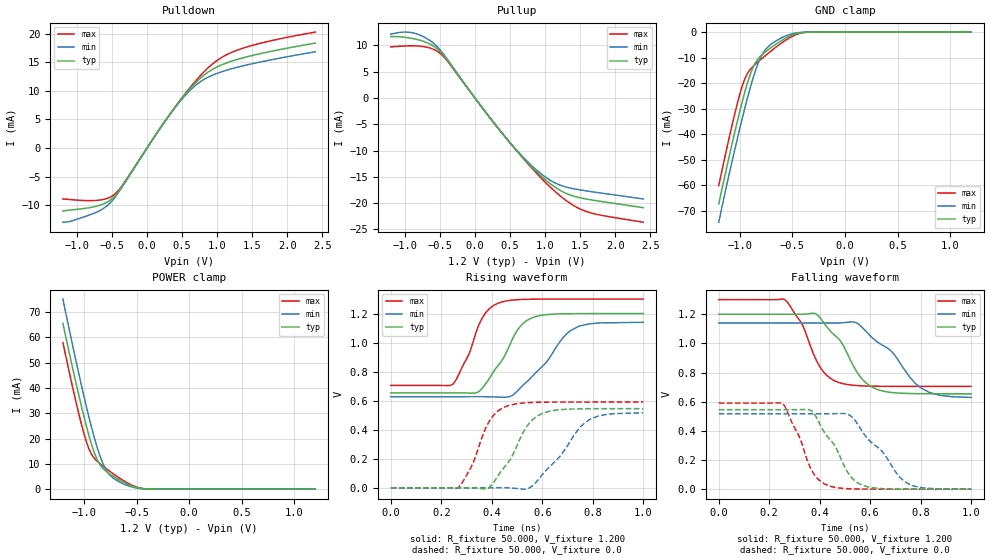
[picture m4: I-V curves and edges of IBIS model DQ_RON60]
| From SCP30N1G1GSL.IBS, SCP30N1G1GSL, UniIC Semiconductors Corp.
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|   Model DQ_RON60
[Model] DQ_RON60
Model_type I/O
Vinl =  0.500V
Vinh =  0.700V
Vmeas =  0.600V
Rref =  50.000
Vref =  0.600V
C_comp   1.373pF   1.353pF   1.403pF
[Model Spec]
Vinh   0.700V   0.670V   0.750V
Vinl   0.500V   0.470V   0.550V
Vmeas   0.600V   0.570V   0.650V
Vref   0.600V   0.570V   0.650V
Rref   50.000   NA   NA
[Temperature Range]   25.000   85.000   -40.000
[Voltage Range]   1.200V   1.140V   1.300V
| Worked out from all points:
|   slope of the pulldown table from 0 to 0.18 V, typ, clamps not added: 53.9 ohm
|   slope of the pullup table from 0 to 0.18 V, typ, clamps not added: 56.5 ohm
|   GND clamp passes 1 mA (typ) near -0.49 V on its own axis
|   POWER clamp passes 1 mA (typ) near -0.53 V on its own axis
|   rising waveform, R_fixture 50.000, V_fixture 1.200: 20-80 % time 110ps typ, 145ps min, 85.5ps max; typ from 0.654 V to 1.2 V
|   rising waveform, R_fixture 50.000, V_fixture 0.0: 20-80 % time 110ps typ, 142ps min, 85.3ps max; typ from 0 V to 0.545 V
|   falling waveform, R_fixture 50.000, V_fixture 1.200: 20-80 % time 125ps typ, 167ps min, 96.1ps max; typ from 1.2 V to 0.654 V
|   falling waveform, R_fixture 50.000, V_fixture 0.0: 20-80 % time 110ps typ, 145ps min, 86.1ps max; typ from 0.545 V to 0 V
[Pulldown]
|Voltage   I(typ)   I(min)   I(max)
-1.2V     -11mA      -12.97mA   -8.906mA
-719mV    -10.17mA   -11.21mA   -9.16mA
-571mV    -9.478mA   -10.12mA   -8.824mA
-460mV    -8.406mA   -8.674mA   -8.076mA
-349mV    -6.601mA   -6.687mA   -6.475mA
317mV     5.745mA    5.716mA    5.735mA
576mV     9.845mA    9.607mA    9.994mA
761mV     12.21mA    11.59mA    12.66mA
1.02V     14.3mA     13.14mA    15.49mA
1.279V    15.45mA    14.09mA    17.07mA
1.723V    16.78mA    15.31mA    18.63mA
2.4V      18.34mA    16.82mA    20.27mA
[Pullup]
|Voltage   I(typ)   I(min)   I(max)
-1.2V     11.68mA    12.13mA    9.732mA
-1.004V   11.56mA    12.54mA    9.897mA
-819mV    11.12mA    12.15mA    9.898mA
-634mV    10.21mA    10.87mA    9.478mA
-486mV    8.716mA    8.99mA     8.386mA
69mV      -1.235mA   -1.243mA   -1.218mA
439mV     -7.546mA   -7.529mA   -7.523mA
772mV     -12.6mA    -12.39mA   -12.76mA
1.031V    -15.85mA   -15.28mA   -16.4mA
1.29V     -18.09mA   -16.91mA   -19.4mA
1.549V    -19.12mA   -17.59mA   -21.4mA
2.4V      -20.87mA   -19.22mA   -23.63mA
[GND_clamp]
|Voltage   I(typ)   I(min)   I(max)
-1.2V     -67.26mA   -74.42mA   -60.1mA
-1.05V    -39.62mA   -46.47mA   -32.4mA
-1V       -31.05mA   -37.77mA   -24.37mA
-950mV    -23.16mA   -29.46mA   -18.1mA
-925mV    -19.62mA   -25.5mA    -16.02mA
-875mV    -13.89mA   -18.21mA   -13.48mA
-825mV    -10.4mA    -12.16mA   -11.61mA
-775mV    -8.365mA   -7.964mA   -9.852mA
-700mV    -6.001mA   -4.671mA   -7.319mA
-525mV    -1.587mA   -933.3uA   -2.208mA
-375mV    -90.13uA   -49.22uA   -132.9uA
1.2V      0A         0A         0A
[POWER_clamp]
|Voltage   I(typ)   I(min)   I(max)
-1.2V     65.51mA    75.11mA    57.91mA
-1.05V    37.38mA    45.87mA    29.99mA
-1V       28.74mA    36.73mA    21.95mA
-950mV    20.85mA    28.08mA    15.65mA
-925mV    17.34mA    24.01mA    13.56mA
-875mV    11.74mA    16.61mA    11.06mA
-825mV    8.457mA    10.65mA    9.317mA
-775mV    6.603mA    6.7mA      7.708mA
-725mV    5.177mA    4.492mA    6.178mA
-550mV    1.336mA    943.1uA    1.707mA
-400mV    85.95uA    67.55uA    91.19uA
1.2V      0A         0A         0A
[Ramp]
| variable   typ   min   max
dV/dt_r   0.327/0.110n   0.310/0.142n   0.354/85.039p
dV/dt_f   0.328/0.125n   0.307/0.167n   0.357/96.296p
R_load = 50.000
[Rising Waveform]
R_fixture= 50.000
V_fixture= 1.200
V_fixture_min= 1.140
V_fixture_max= 1.300
|time   V(typ)   V(min)   V(max)
0s        654.1mV    627.7mV    705.1mV
244ps     654.2mV    627.7mV    711.7mV
310ps     652.5mV    627.8mV    923.6mV
346ps     660mV      627.9mV    1.11V
431ps     855.6mV    624.7mV    1.275V
499ps     1.079V     662.3mV    1.295V
564ps     1.174V     774.3mV    1.299V
681ps     1.198V     1.032V     1.3V
746ps     1.2V       1.113V     1.3V
1ns       1.2V       1.14V      1.3V
[Rising Waveform]
R_fixture= 50.000
V_fixture= 0.0
V_fixture_min= 0.0
V_fixture_max= 0.0
|time   V(typ)   V(min)   V(max)
0s        47.48nV    152.1nV    27.71nV
267ps     31.45uV    -632.5nV   1.056mV
319ps     280.2uV    -15.58uV   144.9mV
381ps     -6.83mV    63.71uV    429.5mV
421ps     73.34mV    315.7uV    523.8mV
462ps     167.3mV    -97.25uV   563.9mV
539ps     422.8mV    -7.696mV   586mV
598ps     510.4mV    85.98mV    589.5mV
791ps     544.8mV    473.1mV    590.7mV
1ns       545.3mV    516.4mV    590.8mV
[Falling Waveform]
R_fixture= 50.000
V_fixture= 1.200
V_fixture_min= 1.140
V_fixture_max= 1.300
|time   V(typ)   V(min)   V(max)
0s        1.2V       1.14V      1.3V
262ps     1.2V       1.14V      1.3V
332ps     1.2V       1.14V      1.125V
381ps     1.205V     1.14V      905.1mV
424ps     1.123V     1.14V      787.8mV
478ps     1.026V     1.14V      730.9mV
560ps     772.2mV    1.124V     709.4mV
628ps     684.3mV    1.01V      706.1mV
798ps     655mV      697.9mV    705.1mV
1ns       654.1mV    629.2mV    705.1mV
[Falling Waveform]
R_fixture= 50.000
V_fixture= 0.0
V_fixture_min= 0.0
V_fixture_max= 0.0
|time   V(typ)   V(min)   V(max)
0s        545.3mV    517mV      590.8mV
255ps     545.2mV    517mV      584.2mV
315ps     545.5mV    516.9mV    376.3mV
369ps     535.8mV    516.8mV    126.9mV
435ps     351.6mV    517.2mV    23.93mV
520ps     92.68mV    506.3mV    2.706mV
570ps     26.67mV    392.8mV    747.4uV
719ps     602.2uV    78.27mV    16.12uV
755ps     239uV      33.15mV    6.404uV
1ns       488.1nV    75.13uV    27.61nV
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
